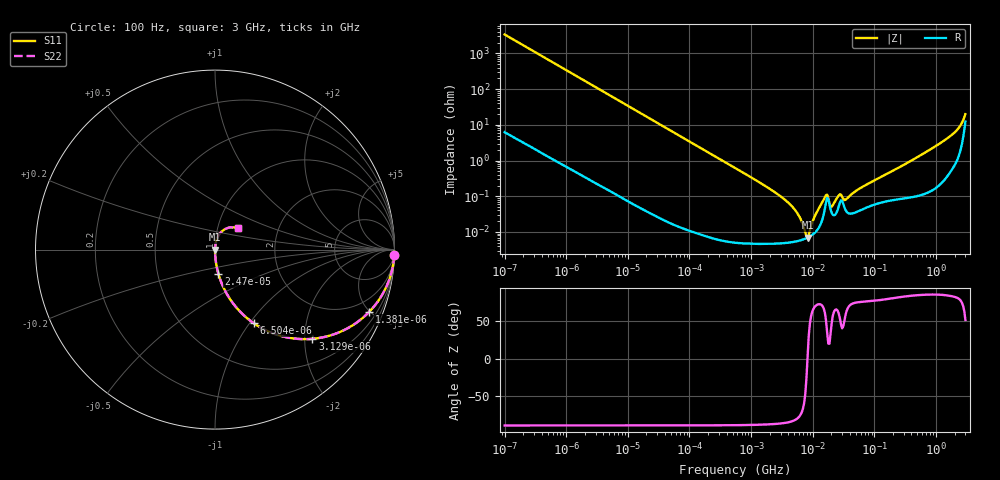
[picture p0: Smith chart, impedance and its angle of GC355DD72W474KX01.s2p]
!Murata Part Number: GC355DD72W474KX01
!These Parameters are Measured in Series Mode Connection
!Data Generated on Jan 08, 2026
!  o--ll--o
!Port1  Port2
!  o------o
!Operation Temp=25[degC], DC Bias Voltage=0[V]
!Freq. Start=100[Hz] Stop=3[GHz] 401[Steps]
# Hz S RI R 50
!Freq.(Hz) S11(Real) S11(Imag) S21(Real) S21(Imag) S12(Real) S12(Imag) S22(Real) S22(Imag)
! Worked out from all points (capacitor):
!   401 points, 100 Hz to 3 GHz, reference 50 ohm
!   read as one part in series: C = 468 nF near 109 Hz
!   lowest |Z| = 6.95 mohm at 8.245 MHz (marker M1)
!   series resonance near 8.21 MHz, so ESL is about 800 pH
!   S11 on the Smith chart (normalised r, x): 100 Hz: 1, -68; 1.381 kHz: 1.01, -4.94; 3.129 kHz: 1.00, -2.18; 6.504 kHz: 1.00, -1.05; 24.7 kHz: 1.00, -0.28; 3 GHz: 1.25, +0.32
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100  0.9991 -0.0294  0.000919 0.0294  0.000919 0.0294  0.9991 -0.0294
432  0.9839 -0.1249  0.0161 0.1249  0.0161 0.1249  0.9839 -0.1249
1381  0.8585 -0.3476  0.1415 0.3476  0.1415 0.3476  0.8585 -0.3476
1788  0.7839 -0.4106  0.2161 0.4106  0.2161 0.4106  0.7839 -0.4106
3129  0.5431 -0.4971  0.4569 0.4971  0.4569 0.4971  0.5431 -0.4971
6504  0.2167 -0.4109  0.7833 0.4109  0.7833 0.4109  0.2167 -0.4109
24699  0.0191 -0.1358  0.9809 0.1358  0.9809 0.1358  0.0191 -0.1358
31977  0.0116 -0.1058  0.9884 0.1058  0.9884 0.1058  0.0116 -0.1058
547723  8.89e-05 -0.00624  0.9999 0.00624  0.9999 0.00624  8.89e-05 -0.00624
3799590  5.01e-05 -0.000717  0.9999 0.000717  0.9999 0.000717  5.01e-05 -0.000717
5361412  5.45e-05 -0.000375  0.9999 0.000375  0.9999 0.000375  5.45e-05 -0.000375
8245314  6.94e-05 3.8e-06  0.9999 -3.8e-06  0.9999 -3.8e-06  6.94e-05 3.8e-06
9794414  8.29e-05 0.000161  0.9999 -0.000161  0.9999 -0.000161  8.29e-05 0.000161
1.572531e7  0.000444 0.000832  0.9996 -0.000832  0.9996 -0.000832  0.000444 0.000832
1.713898e7  0.000902 0.000632  0.9991 -0.000632  0.9991 -0.000632  0.000902 0.000632
2.035898e7  0.000338 0.000382  0.9997 -0.000382  0.9997 -0.000382  0.000338 0.000382
2.635803e7  0.000511 0.000921  0.9995 -0.000921  0.9995 -0.000921  0.000511 0.000921
3.562563e7  0.000366 0.000768  0.9996 -0.000768  0.9996 -0.000768  0.000366 0.000768
1.751444e8  0.000767 0.00451  0.9992 -0.00451  0.9992 -0.00451  0.000767 0.00451
1.573002e9  0.00574 0.043  0.9943 -0.043  0.9943 -0.043  0.00574 0.043
2.219584e9  0.0155 0.0708  0.9845 -0.0708  0.9845 -0.0708  0.0155 0.0708
3e9  0.1268 0.1229  0.8732 -0.1229  0.8732 -0.1229  0.1268 0.1229
